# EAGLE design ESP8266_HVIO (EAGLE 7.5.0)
COPYRIGHT: © 2016 luani.de; LICENSE: CC-BY-SA 4.0; PROJEKT: EPS8266 HV I/O Modul; REVISION: 1.0

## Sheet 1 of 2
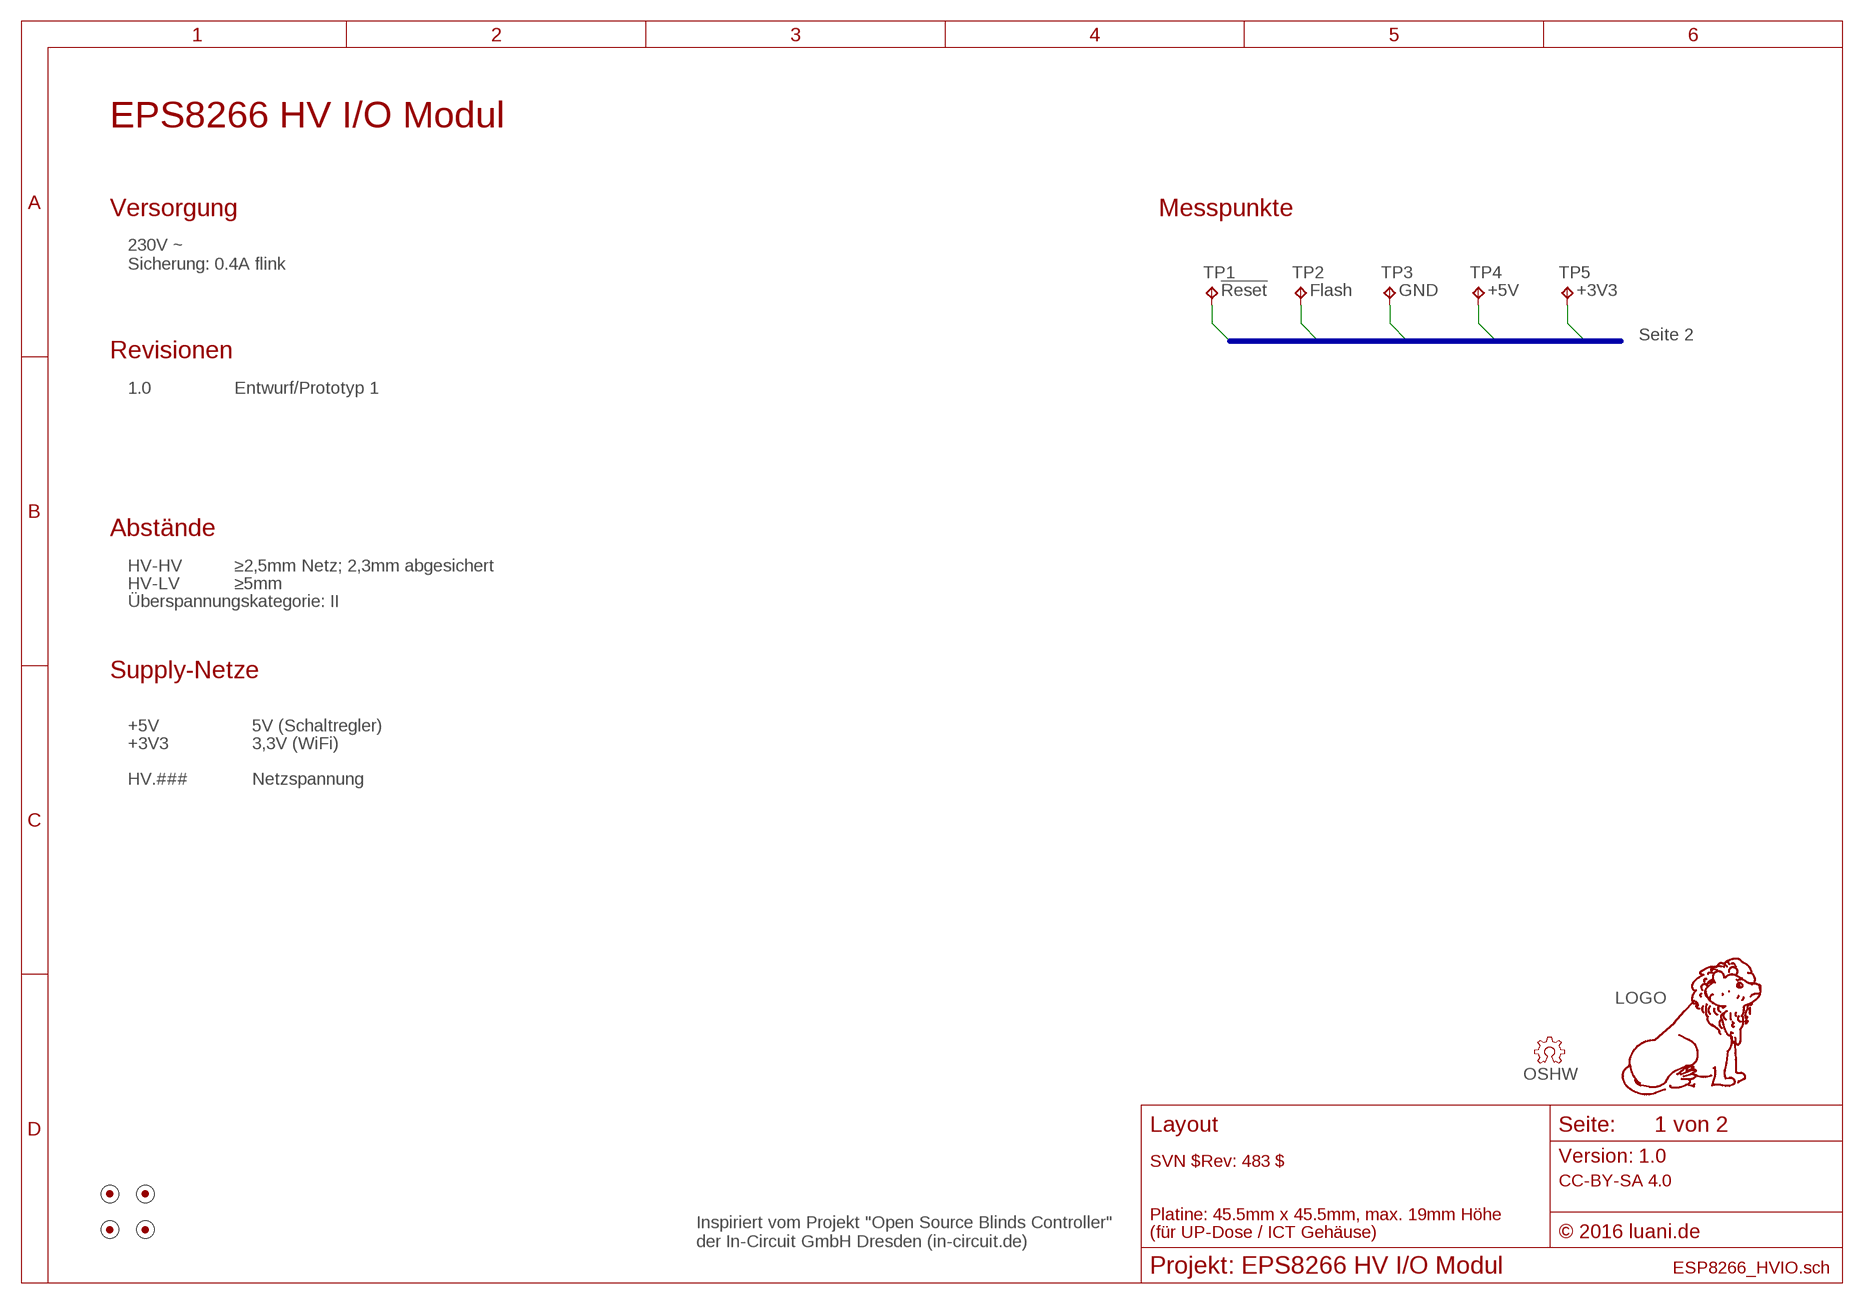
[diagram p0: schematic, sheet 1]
FRAME1 (FRAME_A4-L): TEXT-1: Layout; TEXT-2: SVN $Rev: 483 $; TEXT-4: Platine: 45.5mm x 45.5mm, max. 19mm Höhe; TEXT-5: (für UP-Dose / ICT Gehäuse)

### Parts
LOGO  LOGO-10MM-TPLACE  [10MM-TPLACE]
MARK1  FIDUCIAL-1.0/CREAM  [FIDUCIAL-1MM/CREAM]
MARK2  FIDUCIAL-1.0/CREAM  [FIDUCIAL-1MM/CREAM]
MARK3  FIDUCIAL-1.0/CREAM  [FIDUCIAL-1MM/CREAM]
MARK4  FIDUCIAL-1.0/CREAM  [FIDUCIAL-1MM/CREAM]
OSHW  OSHW-3MM-FILL-TPLACE  [OSHW-FILL-3MM-TPLACE]
TP1  TPTP15R  [TP15R]
TP2  TPTP15R  [TP15R]
TP3  TPTP15R  [TP15R]
TP4  TPTP15R  [TP15R]
TP5  TPTP15R  [TP15R]

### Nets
+3V3: TP5.TP ; also sheet 2
+5V: TP4.TP ; also sheet 2
GND: TP3.TP ; also sheet 2
WIFI.!RST: TP1.TP ; also sheet 2
WIFI.IO#0: TP2.TP ; also sheet 2

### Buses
TEST:WIFI.!RST,WIFI.IO#0,GND,+5V,+3V3

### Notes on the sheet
- Versorgung | Messpunkte
- 230V ~
  Sicherung: 0.4A flink
- Seite 2
- Revisionen
- 1.0 | Entwurf/Prototyp 1
- Abstände
- HV-HV | ≥2,5mm Netz; 2,3mm abgesichert
- HV-LV | ≥5mm
- Überspannungskategorie: II
- Supply-Netze
- +5V | 5V (Schaltregler)
- +3V3 | 3,3V (WiFi)
- HV.### | Netzspannung
- Inspiriert vom Projekt "Open Source Blinds Controller"
  der In-Circuit GmbH Dresden (in-circuit.de)

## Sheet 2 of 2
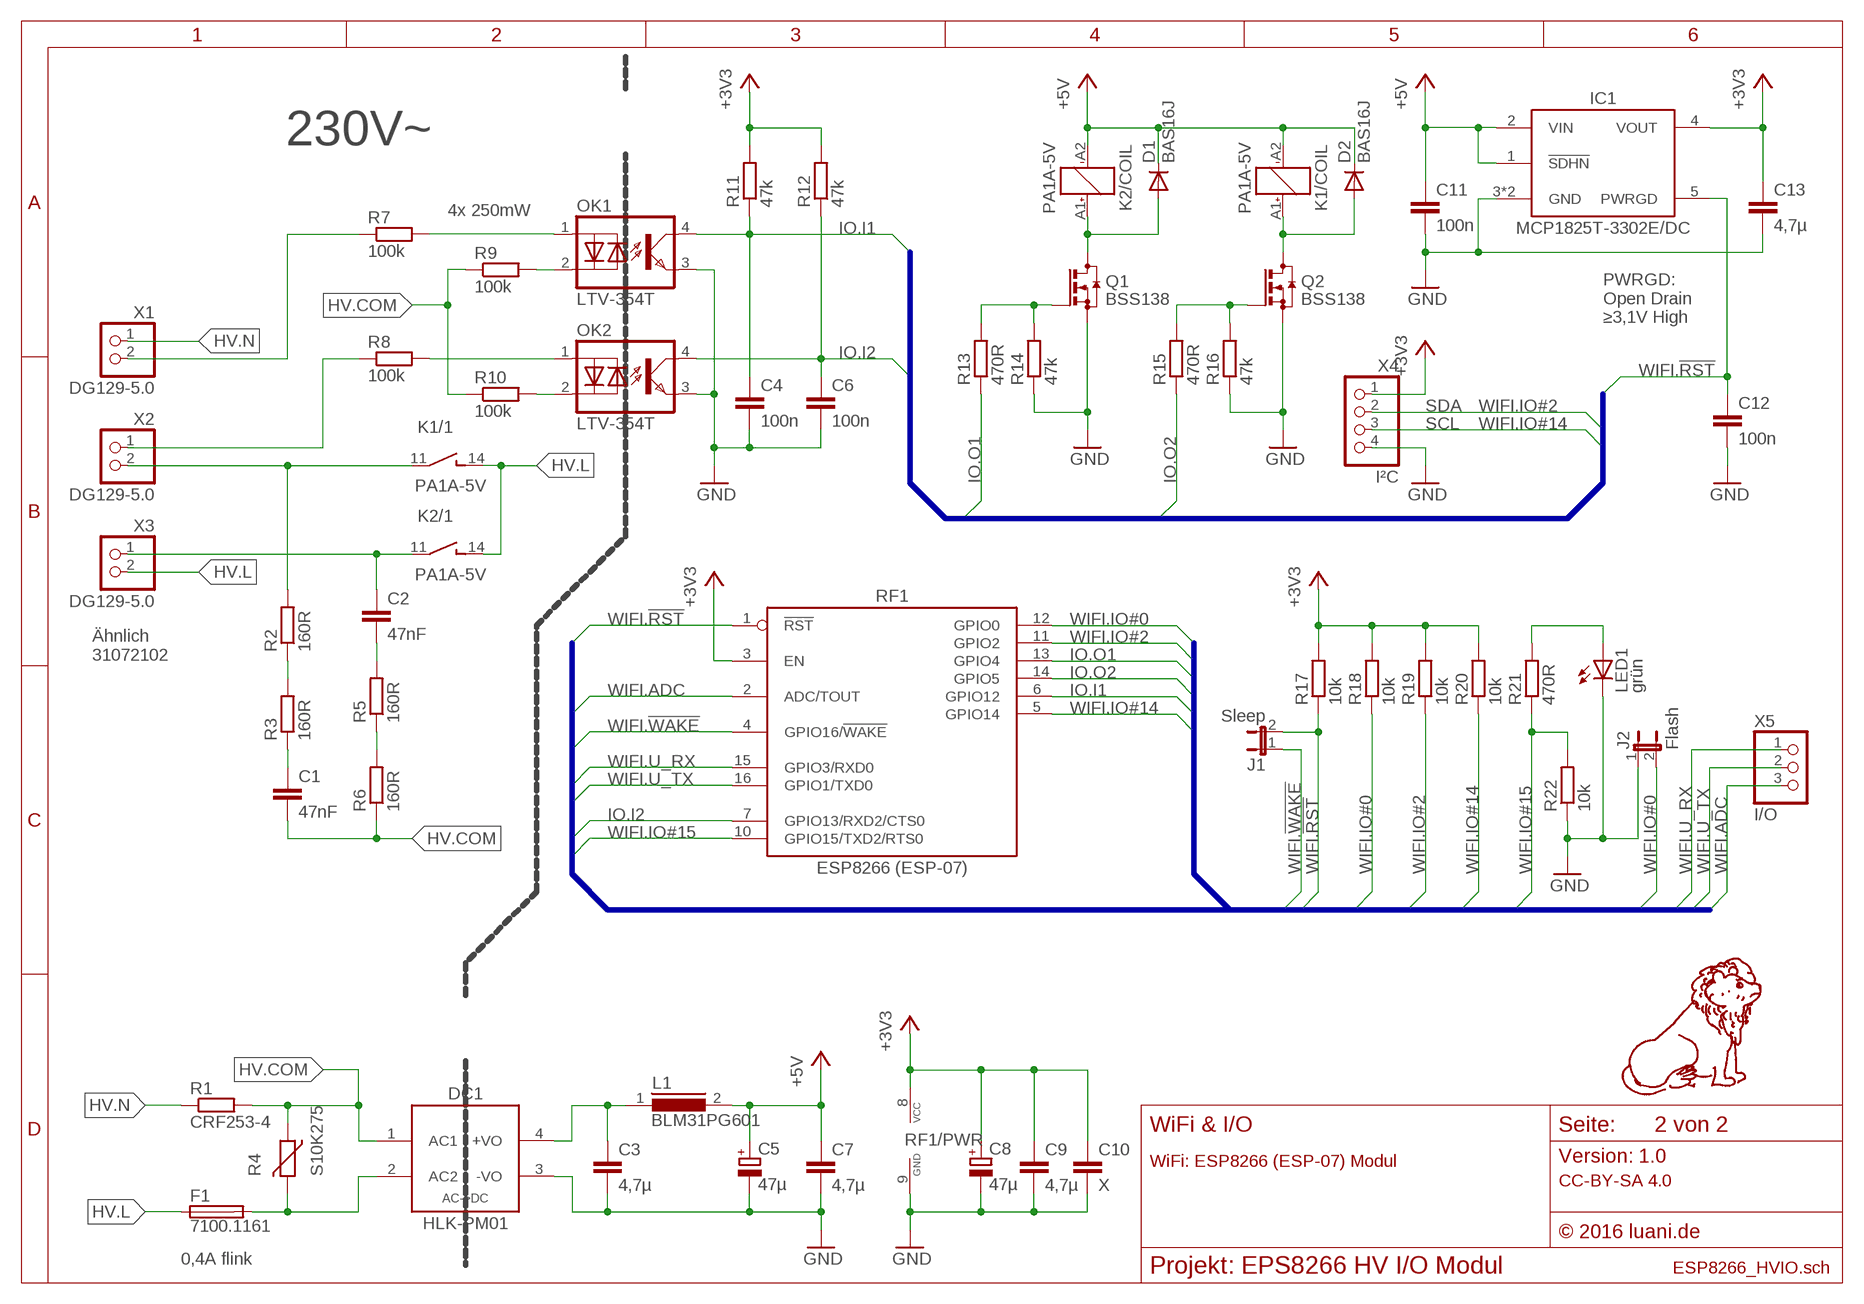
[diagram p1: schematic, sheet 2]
FRAME2 (FRAME_A4-L/LOGO): TEXT-1: WiFi & I/O; TEXT-2: WiFi: ESP8266 (ESP-07) Modul

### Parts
C1  47nF  C_PHE840M-10  [KEMET_PHE840M-10]
C2  47nF  C_PHE840M-10  [KEMET_PHE840M-10]
C3  4,7µ  C-0805  [C-0805]
C4  100n  C-0603  [C-0603]
C5  47µ  CPOL-EUE2-5  [E2-5]
C6  100n  C-0603  [C-0603]
C7  4,7µ  C-0805  [C-0805]
C8  47µ  CPOL-EUE2-5  [E2-5]
C9  4,7µ  C-0805  [C-0805]
C10  X  C-0805  [C-0805]
C11  100n  C-0603  [C-0603]
C12  100n  C-0603  [C-0603]
C13  4,7µ  C-0805  [C-0805]
D1  BAS16J  DIODE-SOD323  [DIODE-SOD323]
D2  BAS16J  DIODE-SOD323  [DIODE-SOD323]
DC1  HLK-PM01  ACDC-S-HLK_PM01  [HLK_PM01]
F1  7100.1161  FUSE-FRT250  [SCHURTER_FRT250]
IC1  MCP1825T-3302E/DC  MCP1825/DC  [SOT-223/5]
J1  Sleep  JUMPER-2-R  [JUMPER-2-R]
J2  Flash  JUMPER-2-R  [JUMPER-2-R]
K1  PA1A-5V  1_SPST-PAN_PA1A  [PAN_PA1A]
K2  PA1A-5V  1_SPST-PAN_PA1A  [PAN_PA1A]
L1  BLM31PG601  INDUCTOR-BLM31  [BLM31P]
LED1  grün  LED-CHIPLED-0603  [CHIPLED-0603]
OK1  LTV-354T  OC-AC_LTV-354  [LITEON_LTV-354]
OK2  LTV-354T  OC-AC_LTV-354  [LITEON_LTV-354]
Q1  BSS138  BSS123  [SOT23]
Q2  BSS138  BSS123  [SOT23]
R1  CRF253-4  R-EU_0414/5V  [0414V]
R2  160R  R-1206  [R-1206]
R3  160R  R-1206  [R-1206]
R4  S10K275  VDR-S10K275  [EPCOS_S10K275]
R5  160R  R-1206  [R-1206]
R6  160R  R-1206  [R-1206]
R7  100k  R-0805  [R-0805]
R8  100k  R-0805  [R-0805]
R9  100k  R-0805  [R-0805]
R10  100k  R-0805  [R-0805]
R11  47k  R-0603  [R-0603]
R12  47k  R-0603  [R-0603]
R13  470R  R-0603  [R-0603]
R14  47k  R-0603  [R-0603]
R15  470R  R-0603  [R-0603]
R16  47k  R-0603  [R-0603]
R17  10k  R-0603  [R-0603]
R18  10k  R-0603  [R-0603]
R19  10k  R-0603  [R-0603]
R20  10k  R-0603  [R-0603]
R21  470R  R-0603  [R-0603]
R22  10k  R-0603  [R-0603]
RF1  ESP8266 (ESP-07)  ESP-07_ESP07  [EXP_ESP07-SMD]
X1  DG129-5.0  1PIN-2-31012102  [31012102]
X2  DG129-5.0  1PIN-2-31012102  [31012102]
X3  DG129-5.0  1PIN-2-31012102  [31012102]
X4  I²C  PINHD-1X4  [1X04]
X5  I/O  PINHD-1X3  [1X03]

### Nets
+3V3: C8.+ C9.1 C10.1 C13.1 IC1.4(VOUT) R11.2 R12.2 R17.2 R18.2 R19.2 R20.2 RF1.3(EN) RF1.8(VCC) X4.1 ; also sheet 1
+5V: C5.+ C7.1 C11.1 D1.C D2.C IC1.1(!SDHN) IC1.2(VIN) K1.A2(/COIL:A2) K2.A2(/COIL:A2) L1.2 ; also sheet 1
GND: C3.2 C4.2 C5.- C6.2 C7.2 C8.- C9.2 C10.2 C11.2 C12.2 C13.2 DC1.3(-VO) IC1.3(GND) IC1.6(GND) J2.1 LED1.C OK1.3(E) OK2.3(E) Q1.2(S) Q2.2(S) R14.1 R16.1 R22.1 RF1.9(GND) X4.4 ; also sheet 1
HV.COM [HV-gesichert]: C1.2 DC1.1(AC1) R1.2 R4.1 R6.1 R9.1 R10.1
HV.IN1 [HV-gesichert]: R7.1 X1.2
HV.IN2 [HV-gesichert]: R8.1 X2.1
HV.L [HV-Netz]: F1.1 K1.14 K2.14 X3.2
HV.N [HV-Netz]: R1.1 X1.1
HV.OUT1 [HV-Netz]: K1.11 R2.2 X2.2
HV.OUT2 [HV-Netz]: C2.1 K2.11 X3.1
IO.I1: C4.1 OK1.4(C) R11.1 RF1.6(GPIO12)
IO.I2: C6.1 OK2.4(C) R12.1 RF1.7(GPIO13/RXD2/CTS0)
IO.O1: R13.1 RF1.13(GPIO4)
IO.O2: R15.1 RF1.14(GPIO5)
N$1: C3.1 DC1.4(+VO) L1.1
N$2 [HV-gesichert]: DC1.2(AC2) F1.2 R4.2
N$3 [HV-gesichert]: C2.2 R5.2
N$11: Q2.1(G) R15.2 R16.2
N$12 [HV-gesichert]: R2.1 R3.2
N$13 [HV-gesichert]: C1.1 R3.1
N$14 [HV-gesichert]: R5.1 R6.2
N$15: Q1.1(G) R13.2 R14.2
N$16 [HV-gesichert]: OK1.2(CA) R9.2
N$17 [HV-gesichert]: OK2.2(CA) R10.2
N$18 [HV-gesichert]: OK1.1(AC) R7.2
N$19 [HV-gesichert]: OK2.1(AC) R8.2
N$20: D2.A K1.A1(/COIL:A1) Q2.3(D)
N$21: D1.A K2.A1(/COIL:A1) Q1.3(D)
N$22: LED1.A R21.2
WIFI.!RST: C12.1 IC1.5(PWRGD) J1.2 R17.1 RF1.1(!RST) ; also sheet 1
WIFI.!WAKE: J1.1 RF1.4(GPIO16/!WAKE)
WIFI.ADC: RF1.2(ADC/TOUT) X5.3
WIFI.IO#0: J2.2 R18.1 RF1.12(GPIO0) ; also sheet 1
WIFI.IO#2: R19.1 RF1.11(GPIO2) X4.2
WIFI.IO#14: R20.1 RF1.5(GPIO14) X4.3
WIFI.IO#15: R21.1 R22.2 RF1.10(GPIO15/TXD2/RTS0)
WIFI.U_RX: RF1.15(GPIO3/RXD0) X5.1
WIFI.U_TX: RF1.16(GPIO1/TXD0) X5.2

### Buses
IO:IO.I1,IO.I2,IO.O1,IO.O2,WIFI.!RST,WIFI.IO#2,WIFI.IO#14
WIFI:WIFI.!RST,WIFI.!WAKE,WIFI.U_RX,WIFI.U_TX,WIFI.ADC,WIFI.IO#0,WIFI.IO#2,WIFI.IO#14,WIFI.IO#15,IO.I1,IO.I2,IO.O1,IO.O2

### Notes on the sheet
- ⚠ 230V~ | ⚡
- 4x 250mW
- PWRGD:
  Open Drain
  ≥3,1V High
- SDA
- SCL
- Ähnlich
  31072102
- ⚡
- 0,4A flink

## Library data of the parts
C1 C2 = luani_rc-tht:C: Capacitor
C3 C4 C6 C7 C9-C13 = luani_rc-smd:C: Capacitor
C5 C8 = rcl:CPOL-EU: POLARIZED CAPACITOR, European symbol
D1 D2 = leo_misc-smd:DIODE: SMD Diode
DC1 = luani_modules:ACDC-S: AC->DC Converter, 1 Out
F1 = luani_protection:FUSE: Fuse
IC1 = luani_chips:MCP1825: Microchip LDO
J1 J2 = leo_misc-smd:JUMPER-2: Jumper
K1 K2 = luani_relay:1_SPST: 1x SPST Relay
L1 = leo_inductor-fastron:INDUCTOR: Fastron SMD Inductor
LED1 = leo_misc-smd:LED: SMD LED
LOGO = leo_misc-logo:LOGO: leo-andres.de PCB Logo
MARK1-MARK4 = leo_misc-logo:FIDUCIAL: Fiducial
OK1 OK2 = luani_misc-smd:OC-AC: Optocoupler, AC Input
OSHW = leo_misc-logo:OSHW: OSHW Logo
Q1 Q2 = transistor-small-signal:BSS123: N-CHANNEL MOS FET
R1 = rcl:R-EU_: RESISTOR, European symbol
R2 R3 R5-R22 = luani_rc-smd:R: Resistor
R4 = luani_protection:VDR: Varistor
RF1 = luani_modules:ESP-07: ESP-8266 ESP07
TP1 = testpad:TP: Test pad; TP_SIGNAL_NAME: !Reset
TP2 = testpad:TP: Test pad; TP_SIGNAL_NAME: Flash
TP3 = testpad:TP: Test pad; TP_SIGNAL_NAME: GND
TP4 = testpad:TP: Test pad; TP_SIGNAL_NAME: +5V
TP5 = testpad:TP: Test pad; TP_SIGNAL_NAME: +3V3
X1-X3 = leo_con-ria:1PIN-2: 1 Pin Header, 2 Pole
X4 = leo_con-pinhead:PINHD-1X4: PIN HEADER
X5 = leo_con-pinhead:PINHD-1X3: PIN HEADER

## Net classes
1 HV-Netz: width 1 mm, clearance 5 mm to class 0, clearance 2.5 mm
2 HV-gesichert: width 0.3 mm, clearance 5 mm to class 0, clearance 2.3 mm to class 1, clearance 2.3 mm

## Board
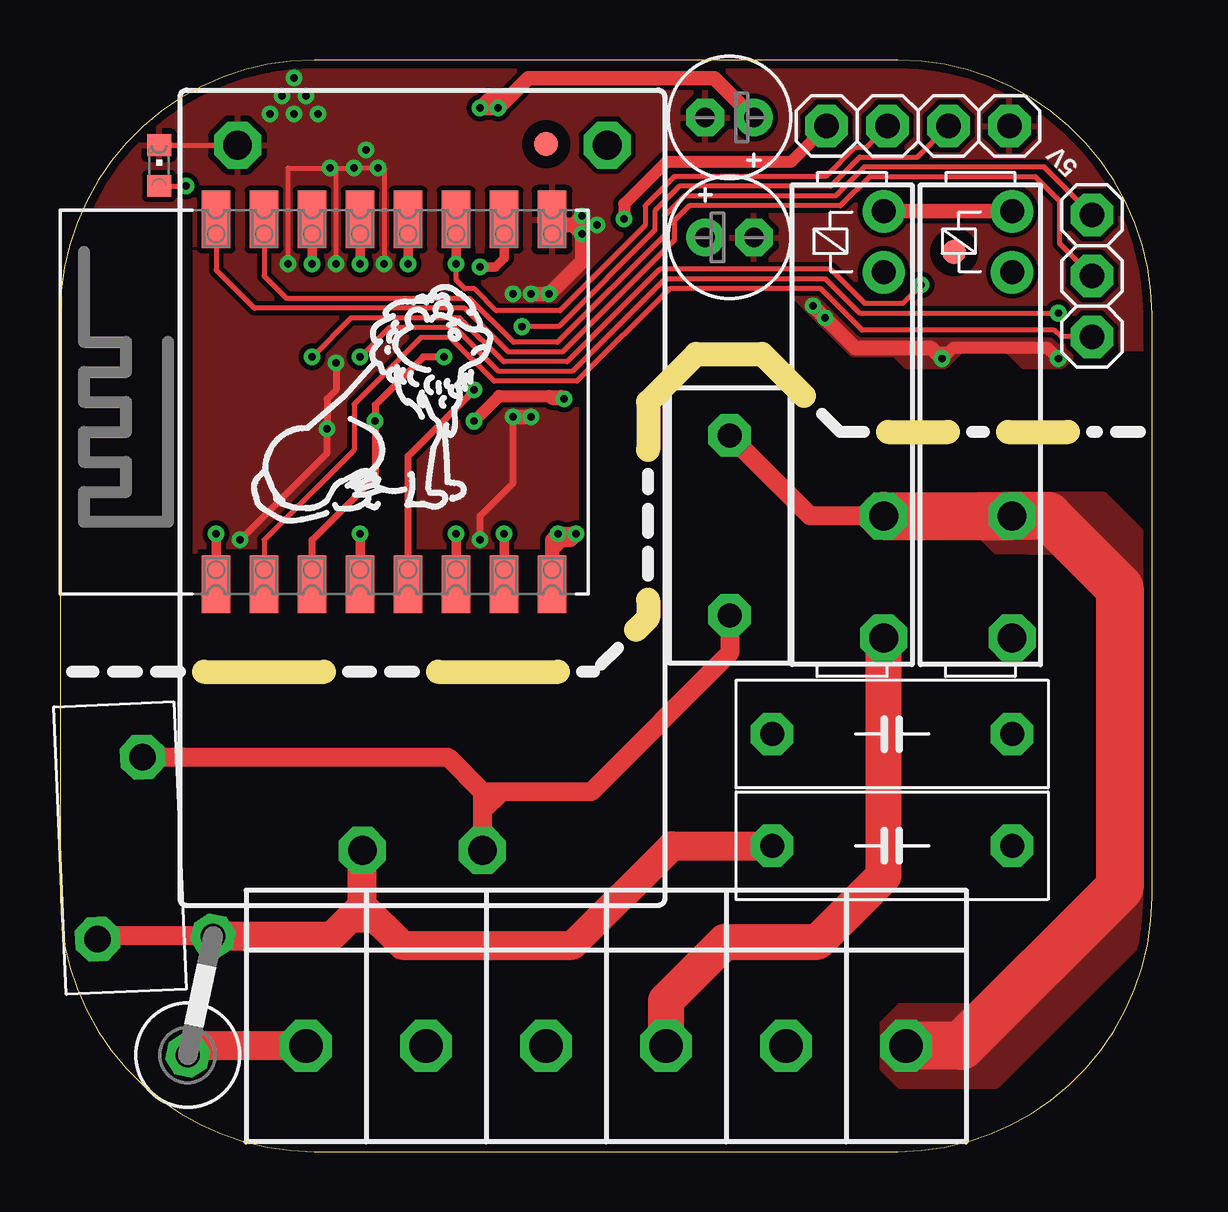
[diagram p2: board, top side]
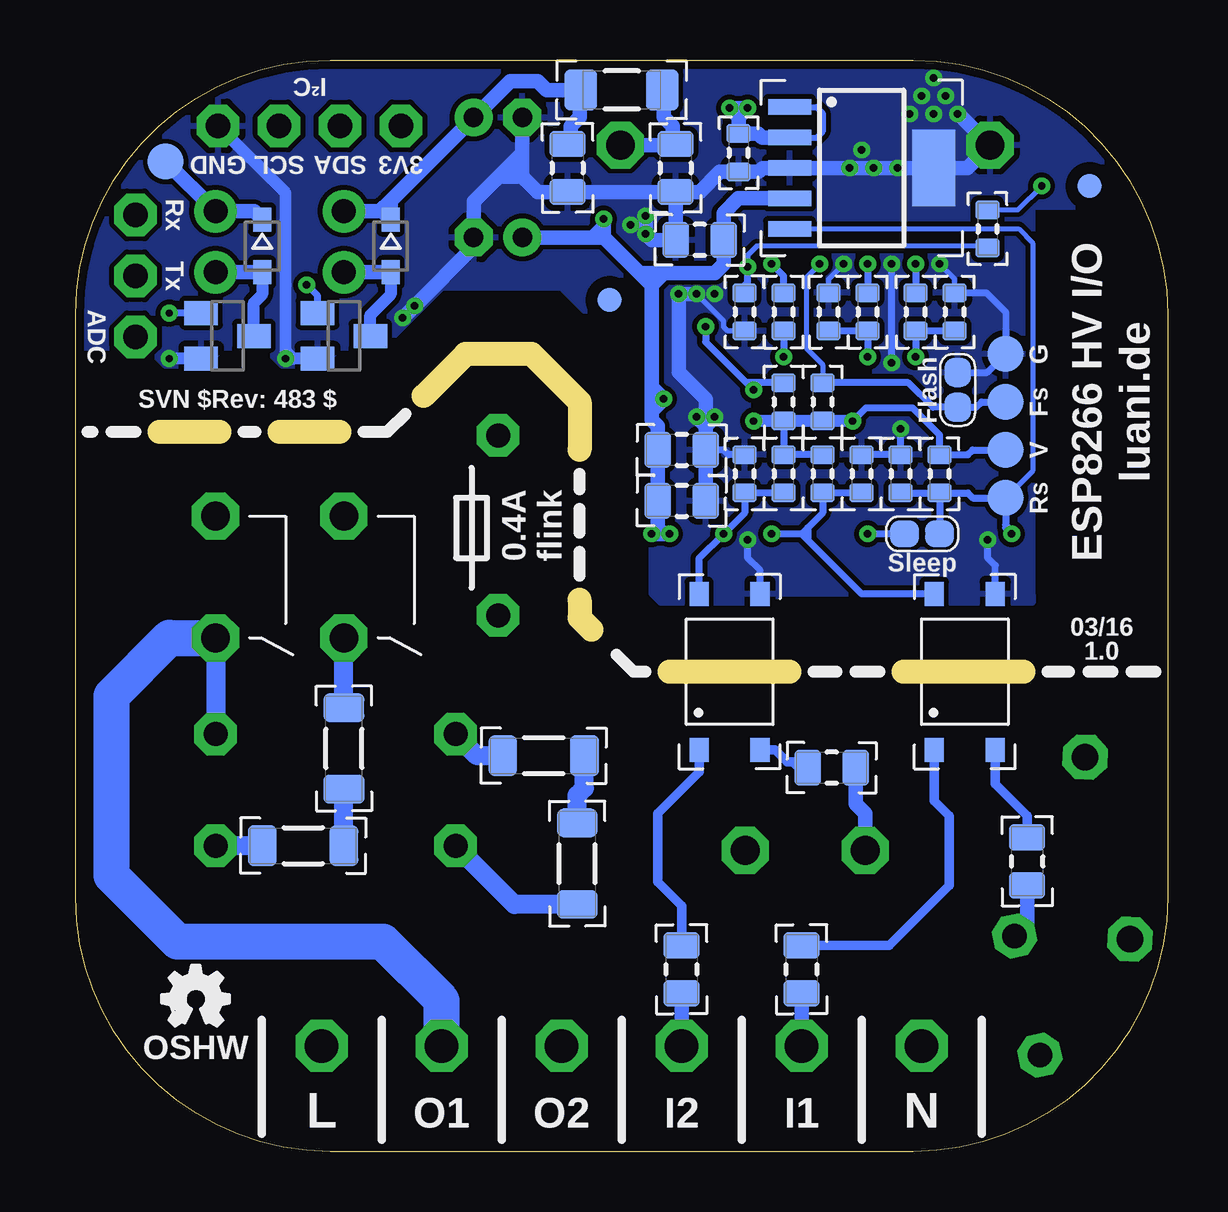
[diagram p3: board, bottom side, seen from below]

Size 45.5 x 45.5 mm. Coordinates in mm from the lower left corner, seen from the top.
Outline: 34.9,45.5 10.6,45.5 arc90 0,34.9 0,10.6 arc90 10.6,0 34.9,0 arc90 45.5,10.6 45.5,34.9 arc90 34.9,45.5
Copper layers (1*16): Top 0.035mm / dielectric 1.5mm / Bottom 0.035mm
Design rules "2-Layer 8x8 *": minimum track width 8mil, minimum drill 0.3mm, track to track 8mil, track to pad 10mil, pad to pad 10mil, via to via 8mil, smd to smd 8mil, copper to edge 0.35mm, drill to drill 0.3mm, minimum pad ring 15mil, minimum via ring 8mil, stop-mask expansion 2.5mil, vias tented up to drill 0.5mm, thermal gap 10mil
Milling: 10 lines

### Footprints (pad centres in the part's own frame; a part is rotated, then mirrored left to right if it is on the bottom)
KEMET_PHE840M-10 = drill 1 octagon: 1 -5,0; 2 5,0
C-0805 = smd 1.1 x 1.5: 1 -1,0; 2 1,0
C-0603 = smd 0.8 x 1: 1 -0.8,0; 2 0.8,0
E2-5 = drill 0.813 pad 1.27: + -1.016,0 | drill 0.813 pad 1.27 octagon: - 1.016,0
DIODE-SOD323 = smd 1 x 0.75: A 1.1,0; C -1.1,0
HLK_PM01 = drill 1.2 octagon: 1 -14.7,2.5; 2 -14.7,-2.5; 3 14.7,7.7; 4 14.7,-7.7
SCHURTER_FRT250 = drill 1 octagon: 1 -3.75,0; 2 3.75,0
SOT-223/5 = smd 0.65 x 1.8: 1 -2.54,-3; 2 -1.27,-3; 3 0,-3; 4 1.27,-3; 5 2.54,-3 | smd 3.2 x 1.8: 6 0,3
JUMPER-2-R = smd 1.2 x 1.1: 1 -0.727,0; 2 0.727,0
PAN_PA1A = drill 1.2 octagon: 11 8.89,1.32; 14 3.81,1.32 | drill 1: A1 -6.35,1.32; A2 -8.89,1.32
BLM31P = smd 1.35 x 1.7: 1 -1.7,0; 2 1.7,0
CHIPLED-0603 = smd 0.9 x 1: A 0.85,0; C -0.85,0
FIDUCIAL-1MM/CREAM = smd 1 x 1: FIDUCIAL 0,0
LITEON_LTV-354 = smd 1 x 0.8: 1 -3.25,1.27; 2 -3.25,-1.27; 3 3.25,-1.27; 4 3.25,1.27
SOT23 = smd 1 x 1.4: 1 -0.95,-1.1; 2 0.95,-1.1; 3 0,1.1
0414V = drill 1.016 octagon: 1 -2.54,0; 2 2.54,0
R-1206 = smd 1.2 x 1.7: 1 -1.7,0; 2 1.7,0
EPCOS_S10K275 = drill 1.1 octagon: 1 -3.75,1.1; 2 3.75,-1.1
R-0805 = smd 1.1 x 1.5: 1 -1,0; 2 1,0
R-0603 = smd 0.8 x 1: 1 -0.8,0; 2 0.8,0
EXP_ESP07-SMD = smd 2.4 x 1.2: 1 -7.6,4.5; 2 -7.6,2.5; 3 -7.6,0.5; 4 -7.6,-1.5; 5 -7.6,-3.5; 6 -7.6,-5.5; 7 -7.6,-7.5; 8 -7.6,-9.5; 9 7.6,-9.5; 10 7.6,-7.5; 11 7.6,-5.5; 12 7.6,-3.5; 13 7.6,-1.5; 14 7.6,0.5; 15 7.6,2.5; 16 7.6,4.5
TP15R = smd 1.5 x 1.5: TP 0,0
31012102 = drill 1.4 octagon: 1 4,2.5; 2 4,-2.5
1X04 = drill 1.016 octagon: 1 -3.81,0; 2 -1.27,0; 3 1.27,0; 4 3.81,0
1X03 = drill 1.016 octagon: 1 -2.54,0; 2 0,0; 3 2.54,0

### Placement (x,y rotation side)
C1  34.67,12.75 180 top
C2  34.67,17.4 180 top
C3  20.5,41 270 bottom
C4  12.75,28.25 90 bottom
C5  27.9,43.1 180 top
C6  17.62,28.25 90 bottom
C7  25,41 270 bottom
C8  27.9,38.1 0 top
C9  20.25,27.12 0 bottom
C10  20.25,29.25 0 bottom
C11  17.88,41.63 270 bottom
C12  11.12,28.25 90 bottom
C13  19.5,38 180 bottom
D1  37.73,37.75 270 bottom
D2  32.38,37.75 270 bottom
DC1  15.1,27.25 90 top
F1  27.9,26.1 270 top
IC1  12.75,41 270 bottom
J1  10.23,25.75 0 bottom
J2  8.75,31.75 270 bottom
K1  33,30.3 270 top
K2  38.35,30.3 270 top
L1  22.75,44.25 180 bottom
LED1  4.12,41.1 270 top
LOGO  13,31.25 0 top
MARK1  20.25,42 0 top
MARK2  3.25,40.25 0 bottom
MARK3  37.25,37.5 0 top
MARK4  23.25,35.5 0 bottom
OK1  8.45,20 90 bottom
OK2  18.25,20 90 bottom
OSHW  40.5,6.5 0 bottom
Q1  39.17,34 270 bottom
Q2  34.32,34 270 bottom
R1  5.85,6.5 78 top
R2  34.32,16.8 90 bottom
R3  36.02,12.75 0 bottom
R4  2.5,12.65 92.5 top
R5  26,16.5 180 bottom
R6  24.6,12 90 bottom
R7  15.25,7.6 90 bottom
R8  20.25,7.6 90 bottom
R9  5.85,12.1 90 bottom
R10  14,16 180 bottom
R11  14.38,28.25 90 bottom
R12  16,28.25 90 bottom
R13  12.5,35 270 bottom
R14  14.12,35 270 bottom
R15  10.5,35 270 bottom
R16  8.88,35 270 bottom
R17  9.5,28.25 90 bottom
R18  14.38,31.25 270 bottom
R19  16,35 270 bottom
R20  16,31.25 270 bottom
R21  7.5,38.46 90 bottom
R22  17.62,35 90 bottom
RF1  11,31.25 90 top
TP1  6.75,27.25 0 bottom
TP2  6.75,31.25 0 bottom
TP3  6.75,33.25 0 bottom
TP4  41.75,41.27 0 bottom
TP5  6.75,29.25 0 bottom
X1  12.75,0.4 90 top
X2  22.75,0.4 90 top
X3  32.75,0.4 90 top
X4  35.75,42.75 0 top
X5  43,36.5 270 top

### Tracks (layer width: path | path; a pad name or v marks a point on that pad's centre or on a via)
+3V3  (via drill 0.3)
  Top 0.3: RF1.3 10.5,25.5 13.12,28.12 v13.12,30.45 13.12,31.12 15.12,33.12 v16,33.12
  Top 0.5: X4.1 30.44,41.25 25.25,41.25 23.5,39.5 v23.5,38.88 | v17.25,30.45 18.3,31.5 20.38,31.5 | 20.38,31.5 20.5,31.38 v21,31.38 20.88,31.5 20.38,31.5
  Top 0.6: RF1.8 20.5,25.12 | 20.5,25.12 20.5,25.5 v20.75,25.75 v21.5,25.75 21.25,25.5 20.88,25.5 20.5,25.12
  Bottom 0.3: R20.2 R12.2 R11.2 | R19.2 v16,33.12 | v13.12,30.45 12.57,31 10.62,31 9.5,29.88 R17.2 8.32,29.05 8.12,29.25 TP5.TP
  Bottom 0.5: v17.25,30.45 R20.2 R18.2 v13.12,30.45
  Bottom 0.6: 22,36.62 18.88,36.62 18.5,37 C13.1 18.5,39.12 17.89,39.73 IC1.4 | v20.75,25.75 v21.5,25.75 21.25,26 | 22,36.62 23.48,38.1 | 23.48,38.1 23.95,38.1 | 23.95,38.1 C8.+ | v23.5,38.88 23.5,38.12 23.48,38.1 | 23.95,38.1 23.5,38.55 | 22,36.62 21.5,36.12 | 21.5,36.12 21.5,31.88 | 21.5,36.12 21,36.62 | 21.5,31.88 v21,31.38 21.5,30.88 | 21.5,31.88 21.5,30.88 | 21.5,30.88 21.5,30.5 21.25,30.25 C10.1 C9.1 21.25,26 | 21.25,26 21,25.75
+5V  (via drill 0.3)
  Top 0.6: C5.+ 27.27,44.75 19.5,44.75 v18.25,43.5 v17.5,43.5 17.88,43.88 18.5,43.88 | K1.A2 K2.A2
  Bottom 0.25: IC1.2 14.62,42.27 14.38,42.52 14.38,43.29 14.62,43.54 IC1.1
  Bottom 0.6: 32.72,39.19 D2.C 32.38,39.64 | TP4.TP K2.A2 38.06,39.19 D1.C | 32.38,39.64 C5.+ 27.39,44.62 26.25,44.62 25.88,44.25 L1.2 24.5,44.25 24.5,43.12 24.88,42.75 24.88,42 C7.1 | 32.38,39.64 32.83,39.19 K1.A2 | IC1.2 16.89,42.27 17.06,42.44 C11.1 17.88,43.12 | 17.88,43.12 v18.25,43.5 v17.5,43.5 17.88,43.12
GND  (via drill 0.3)
  Top 0.203: v9.5,37 9.5,41 11.5,41 | v13.5,37 13.5,41 v12.25,41 11.5,41 | LED1.C DC1.3 | v11.5,37 11.5,41
  Top 0.3: v17.5,25.5 17.5,26.5 18.88,27.88 v18.88,30.62 | v11.5,32.88 11.5,31.75 11.12,31.38 v11.12,30.12 11.12,29.12 v7.5,25.5
  Top 0.5: v41.6,33.05 41.15,33.5 37.2,33.5 36.99,33.29 | 36.99,33.29 v36.75,33.05 | 36.99,33.29 36.54,33.29
  Top 0.6: v21.75,38.25 v21.75,39 21.38,38.62 | v31.38,35.25 33.12,33.5 36.3,33.5 v36.75,33.05 | v19.62,35.75 v20.38,35.75 21.75,37.12 v21.75,38.25 | RF1.9 20.5,38.62 21.38,38.62 | 21.38,38.62 v21.75,38.25 | v19.62,30.62 v18.88,30.62
  Bottom 0.203: R22.1 18.32,34.2 18.5,34.38 18.5,34.62 v19.62,35.75 | R16.1 8.88,36.38 v9.5,37 | R14.1 14.12,36.38 v13.5,37
  Bottom 0.3: OK2.3 16.98,24.23 17.5,24.75 v17.5,25.5 | C6.2 18.3,29.05 18.5,29.25 C10.2 | R16.1 7.55,35.8 6.75,35 TP3.TP 7.52,32.48 J2.1 | OK1.3 7.18,24.43 7.5,24.75 v7.5,25.5 | C4.2 C12.2 v11.12,30.12 | v11.5,32.88 v11.5,37
  Bottom 0.5: Q2.2 36.42,33.05 | 36.42,33.05 v36.75,33.05 36.75,33.38 | Q1.2 v41.6,33.05 | 36.75,33.38 36.75,39.94 X4.4 | 36.42,33.05 36.75,33.38
  Bottom 0.6: C5.- 26.88,41.62 | 26.88,41.62 28.92,39.58 C8.- 28.92,37.71 v31.38,35.25 v31.88,34.75 | C3.2 C7.2 26.25,40 26.88,40.63 | 26.88,41.62 26.88,40.63 | v21.75,39 v21.75,38.25 21.5,38 C13.2 C3.2 | 26.88,40.63 27.87,40.63 | C9.2 C10.2 19.25,30.25 | v19.62,35.75 v20.38,35.75 20.38,32.5 19.25,31.38 19.25,30.25 | C3.2 19.5,40 18.66,40.84 C11.2 17.04,40.84 16.88,41 IC1.3 IC1.6 8.35,41 DC1.3 8.7,43.25 v8.75,43.25 | 19.25,30.25 v18.88,30.62 v19.62,30.62 19.25,30.25
  other vias: 13.25,41 12.75,41.75 9.75,43.25 10.75,43.25 9.25,44 10.25,44 9.75,44.75 11.25,41 18.88,35.75 22.38,38.62
  pour Bottom (no thermals): 8.38,39 13.75,39 13.75,45 8.38,45
  pour Bottom (rank 6): 0,23.25 5.62,23.25 5.62,22.88 12.88,22.88 13.25,23.25 16.12,23.25 16.5,22.88 21.12,22.88 21.5,23.25 21.5,32.25 25.25,36 30.25,36 32.75,33.5 34.5,33.5 35.25,32.75 36.88,32.75 37.62,33.5 39.38,33.5 40.12,32.75 41.75,32.75 42.5,33.5 45.5,33.5 45.5,34.9 arc90 34.9,45.5 10.6,45.5 arc90 0,34.9
  pour Top (rank 6): 0,23.25 5.62,23.25 5.62,25.25 21,25.25 21.5,25.75 21.5,32.25 25.25,36 30.25,36 33,33.25 34.75,33.25 35.25,32.75 36.88,32.75 37.62,33.5 39.38,33.5 40.12,32.75 41.75,32.75 42.5,33.5 45.5,33.5 45.5,34.9 arc90 34.9,45.5 10.6,45.5 arc90 0,34.9
HV.COM
  Top 0.8: R1.2 1.69,8.98 R4.1
  Top 1.2: C1.2 25.5,12.75 21.35,8.6 14.25,8.6 12.6,10.25 | 12.6,10.25 DC1.1 | R1.2 11.33,8.98 12.09,9.74 | 12.09,9.74 12.6,10.25 | 12.09,9.74 12.99,9.74
  Bottom 0.6: DC1.1 12.6,14.1 13,14.5 R10.1 | R9.1 5.85,9.51 R1.2
  Bottom 0.8: R6.1 27.22,10.3 C1.2
HV.IN1
  Bottom 0.6: R7.1 X1.2
HV.IN2
  Bottom 0.6: R8.1 X2.1
HV.L
  Top 0.8: K1.14 31.26,26.49 F1.1
  Top 2: K1.14 K2.14 41.16,26.49 44.15,23.5 44.15,11 37.55,4.4 X3.2
  pour Top (no thermals): 39,2.7 35,2.7 34.25,3.45 34.25,5.35 35,6.1 38.1,6.1 43.25,11.25 45.05,11.25 45.05,8.75
  pour Top (no thermals): 45.05,23 45.05,25.84 43.5,27.39 38.25,27.39 38.25,25.75 39,25 41.5,25 43.5,23
HV.N
  Top 1.2: X1.1 5.71,4.4 R1.1
HV.OUT1
  Top 1.5: X2.2 25.25,6.3 27.7,8.75 31.57,8.75 34.32,11.5 K1.11
  Bottom 0.8: R2.2 K1.11
HV.OUT2
  Bottom 0.8: K2.11 C2.1
  Bottom 1.5: X3.1 30.25,6.3 32.7,8.75 41.25,8.75 44,11.5 44,19 41.59,21.41 K2.11
IO.I1  (via drill 0.3)
  Top 0.4: RF1.6 v16.5,25.75
  Bottom 0.3: C4.1 R11.1 14.38,26.62 15,26 | 15,26 15.25,25.75 | 15.25,25.75 v16.5,25.75 | OK1.4 12.75,23.25 15,25.5 | 15,25.5 15.25,25.75 | 15,26 15,25.5
IO.I2  (via drill 0.3)
  Top 0.4: RF1.7 v18.5,25.75
  Bottom 0.3: OK2.4 19.52,24.73 v18.5,25.75 17.62,26.62 C6.1 R12.1
IO.O1  (via drill 0.3)
  Top 0.4: RF1.13 v12.5,37
  Bottom 0.3: v12.5,37 R13.1
IO.O2  (via drill 0.3)
  Top 0.4: RF1.14 v10.5,37
  Bottom 0.3: v10.5,37 R15.1
N$1
  Bottom 0.6: DC1.4 20.5,41.95 C3.1 20.62,42 20.62,42.75 21,43.12 21,44.25 L1.1
N$2
  Top 0.8: F1.2 27.9,20.77 22.12,15 17.6,15 | R4.2 16.16,16.44 17.6,15 | 17.6,15 17.6,14.22 | 17.6,14.22 DC1.2 | 17.6,14.22 18.38,15
N$3
  Bottom 0.8: R5.2 28.77,16.5 C2.2
N$11  (via drill 0.3)
  Top 0.203: v35.88,36.12 35.11,35.36 33.53,35.36 32.11,36.78 24.99,36.78 21.13,32.92 18.49,32.92 16.66,34.75 12.12,34.75 v10.5,33.12
  Bottom 0.3: Q2.1 35.42,35.67 v35.88,36.12 | R16.2 R15.2 v10.5,33.12
N$12
  Bottom 0.8: R3.2 R2.1
N$13
  Bottom 0.8: R3.1 C1.1
N$14
  Bottom 0.8: R5.1 24.3,15.15 24.6,14.85 R6.2
N$15  (via drill 0.3)
  Top 0.203: v41.6,34.95 33.33,34.95 31.9,36.37 25.2,36.37 21.34,32.51 18.29,32.51 16.46,34.34 13.72,34.34 v12.5,33.12 | v41.6,34.95
  Bottom 0.3: Q1.1 v41.6,34.95 | R14.2 R13.2 v12.5,33.12
N$16
  Bottom 0.4: R9.2 5.85,14 7.18,15.33 OK1.2
N$17
  Bottom 0.4: OK2.2 16.35,16.75 15.85,16.25 15.62,16.25 | R10.2 15,16.25 15.62,16.25 | 15.62,16.25 15.25,15.88
N$18
  Bottom 0.4: R7.2 11.6,8.6 9.1,11.1 9.1,14 9.72,14.62 OK1.1
N$19
  Bottom 0.4: R8.2 20.25,10.25 21.25,11.25 21.25,14.1 19.52,15.83 OK2.1
N$20
  Bottom 0.5: Q2.3 33.22,34.88 32.38,35.72 D2.A
  Bottom 0.6: D2.A K1.A1
N$21
  Bottom 0.5: Q1.3 38.07,35.38 37.73,35.72 D1.A
  Bottom 0.6: K2.A1 D1.A
N$22  (via drill 0.3)
  Top 0.203: LED1.A v5.25,40.25
  Bottom 0.203: R21.2 6.24,39.26 v5.25,40.25
WIFI.!RST  (via drill 0.3)
  Top 0.4: RF1.1 v6.5,25.75
  Bottom 0.203: IC1.5 6.21,38.46 5.62,37.88 5.62,28.38 TP1.TP
  Bottom 0.3: C12.1 R17.1 | R17.1 8.32,27.45 8.12,27.25 TP1.TP 6.75,26.12 | R17.1 J1.2 | 6.75,26.12 6.75,26 v6.5,25.75 6.5,25.88 6.75,26.12
WIFI.!WAKE  (via drill 0.3)
  Top 0.4: RF1.4 v12.5,25.75
  Bottom 0.3: J1.1 v12.5,25.75
WIFI.ADC
  Top 0.203: X5.3 41.71,33.96 41.43,34.24 33.43,34.24 31.7,35.97 25.4,35.97 21.54,32.11 18.09,32.11 16.26,33.93 15.04,33.93 12.25,31.15 12.25,29.25 8.5,25.5 RF1.2
WIFI.IO#0  (via drill 0.3)
  Top 0.4: RF1.12 v14.5,37
  Bottom 0.203: v14.5,37 15.06,36.44 15.06,33.5 14.38,32.81 R18.1
  Bottom 0.3: TP2.TP 7.75,31.25 7.98,31.02 J2.2 9.77,31.02 10.8,32.05 R18.1
WIFI.IO#2  (via drill 0.3)
  Top 0.203: X4.2 33.59,41.86 33.12,41.86 31.9,40.64 25.6,40.64 24.38,39.42 24.38,38.61 20.83,35.05 18.19,35.05 17.27,35.97 16.87,35.97 16.5,36.33 v16.5,37
  Top 0.4: RF1.11 v16.5,37
  Bottom 0.3: R19.1 16,36.5 v16.5,37
WIFI.IO#14  (via drill 0.3)
  Top 0.203: X4.3 35.72,41.45 33.33,41.45 32.11,40.23 25.81,40.23 24.79,39.22 24.79,38.41 20.78,34.39 v19.25,34.39
  Top 0.3: RF1.5 14.5,29 v17.25,31.75
  Bottom 0.3: R20.1 16.95,32.05 | 16.95,32.05 v17.25,31.75 19.25,33.75 v19.25,34.39 | 16.95,32.05 17.55,32.05
WIFI.IO#15  (via drill 0.3)
  Top 0.4: RF1.10 18.5,37.25 18.12,36.88 v17.5,36.88
  Bottom 0.203: v17.5,36.88 17.5,37.38 17.12,37.75 7.5,37.75 R21.1
  Bottom 0.3: R22.2 17.5,35.8 17.5,36.25 | 17.5,36.25 v17.5,36.88 | 17.5,36.25 17.75,36
WIFI.U_RX
  Top 0.203: X5.1 40.99,41.05 33.53,41.05 32.31,39.83 26.01,39.83 25.2,39.01 25.2,38.2 20.73,33.73 18.9,33.73 17.07,35.56 9.44,35.56 8.5,36.5 RF1.15
WIFI.U_TX
  Top 0.203: X5.2 41.66,37.84 41.66,39.62 40.64,40.64 33.73,40.64 32.51,39.42 26.21,39.42 25.6,38.81 25.6,38 20.93,33.33 18.69,33.33 16.87,35.15 8.1,35.15 6.5,36.75 RF1.16

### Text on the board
tPlace: 5V
bPlace: I²C | 3V3 | SDA | SCL | GND | Rx | Tx | ADC | G | Flash | luani.de | ESP8266 HV I/O | Fs | SVN $Rev: 483 $ | V | Rs | 0.4A / flink | Sleep | 03/16 | 1.0 | OSHW | N | I1 | I2 | O2 | O1 | L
